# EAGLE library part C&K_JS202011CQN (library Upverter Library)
Sub-Miniature Slide Switches
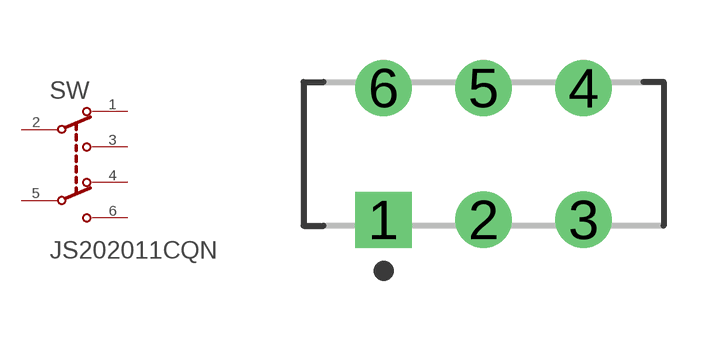
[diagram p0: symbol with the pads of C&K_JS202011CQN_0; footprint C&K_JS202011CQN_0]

Designator prefix SW

## C&K_JS202011CQNC&K_JS202011CQN_0_0 (MF: C&K; MPN: JS202011CQN; centroid_not_specified: No; datasheet: http://www.ckswitches.com/media/1422/js.pdf; digikey_description: SWITCH SLIDE DPDT 300MA 6V; digikey_part_number: 401-2001-ND; lead_free: yes; mouser_part_number: 611-JS202011CQN; package: PTH_DPTD_SW; prefix: SW; rohs: yes; temperature_range_high: +85°C; temperature_range_low: -40°C)  [C&K_JS202011CQN_0]
1  1
2  2
3  3
4  4
5  5
6  6

## Footprint C&K_JS202011CQN_0 (pad centres in mm)
Sub-Miniature Slide Switches
drill 0.9 pad 1.4 square: 1 -2.5,-1.65
drill 0.9 pad 1.4 round: 2 0,-1.65; 3 2.5,-1.65; 4 2.5,1.65; 5 0,1.65; 6 -2.5,1.65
